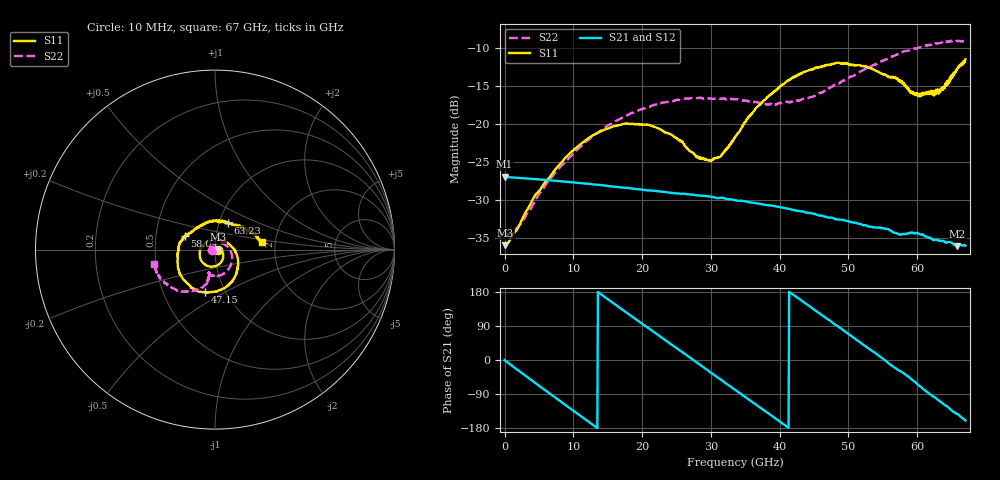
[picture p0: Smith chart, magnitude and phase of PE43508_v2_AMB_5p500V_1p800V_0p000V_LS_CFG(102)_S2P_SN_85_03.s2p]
!Keysight Technologies,N5227A,US51270237,A.10.43.00
!Date: Wednesday, August 22, 2018 17:17:19
!Correction: S11(Full 2 Port(1,3))
!S31(Full 2 Port(1,3))
!S13(Full 2 Port(1,3))
!S33(Full 2 Port(1,3))
!S2P File: Measurements: S11, S31, S13, S33:
# Hz S  dB  R 50
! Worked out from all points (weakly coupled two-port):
!   801 points, 10 MHz to 67 GHz, reference 50 ohm
!   highest |S21| = -26.97 dB at 10 MHz (marker M1); lowest = -36.1 dB at 65.83 GHz (marker M2)
!   lowest |S11| = -36.0 dB at 93.74 MHz (marker M3), VSWR 1.03, Z = 51.6 + j0.019 ohm
!   |S11| at or under -10 dB: start of sweep to end of sweep
!   |S22| runs from -34.5 to -9.1 dB; largest |S21 - S12| = 0.00024
!   S11 on the Smith chart (normalised r, x): 10 MHz: 1.03, -0.00; 47.15 GHz: 0.80, -0.41; 58.04 GHz: 0.70, +0.11; 63.23 GHz: 1.10, +0.34; 67 GHz: 1.70, +0.15
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1e7  -35.87 -1.3  -26.97 -0.2  -26.97 -0.2  -34.46 -179.7
9.37375e7  -35.97 0.7  -26.98 -1.4  -26.99 -1.4  -34.46 177.2
2.35465e9  -32.95 6.0  -27.13 -32.3  -27.13 -32.3  -33.15 120.1
5.871625e9  -27.67 -13.6  -27.37 -79.3  -27.38 -79.3  -28.16 64.4
1.123082e10  -22.54 -59.4  -27.81 -150.0  -27.82 -150.0  -22.86 12.5
1.74274e10  -20.01 -111.5  -28.39 129.2  -28.39 129.2  -19.05 -31.1
2.236791e10  -20.61 -155.5  -28.89 65.3  -28.88 65.2  -17.42 -58.9
2.580115e10  -22.43 166.7  -29.19 21.3  -29.19 21.3  -16.82 -74.8
2.973681e10  -24.83 95.7  -29.55 -29.8  -29.55 -29.8  -16.66 -89.2
3.132782e10  -24.32 62.9  -29.74 -49.9  -29.74 -49.9  -16.72 -94.3
3.3505e10  -21.85 23.8  -30.04 -78.7  -30.05 -78.7  -16.79 -99.9
3.643581e10  -18.10 -13.3  -30.42 -116.2  -30.42 -116.2  -17.14 -104.4
3.88642e10  -16.09 -35.7  -30.76 -147.4  -30.78 -147.4  -17.45 -104.5
4.472582e10  -12.88 -84.1  -31.77 136.8  -31.75 136.8  -16.48 -102.4
4.715421e10  -12.25 -103.0  -32.35 105.8  -32.32 105.7  -15.33 -103.0
5.234594e10  -12.43 -144.1  -33.32 38.2  -33.29 38.0  -12.84 -109.7
5.586291e10  -13.92 -179.4  -33.89 -9.3  -33.89 -9.8  -11.33 -120.5
5.804009e10  -14.63 155.5  -34.49 -35.0  -34.50 -35.6  -10.51 -128.3
6.004979e10  -16.02 122.2  -34.36 -63.9  -34.36 -64.2  -10.09 -135.9
6.323181e10  -15.58 64.4  -35.35 -107.9  -35.38 -108.5  -9.42 -149.8
6.582768e10  -12.75 24.1  -36.08 -142.7  -36.15 -143.1  -9.15 -160.5
6.7e10  -11.53 8.8  -36.00 -159.7  -36.10 -159.9  -9.09 -167.0
